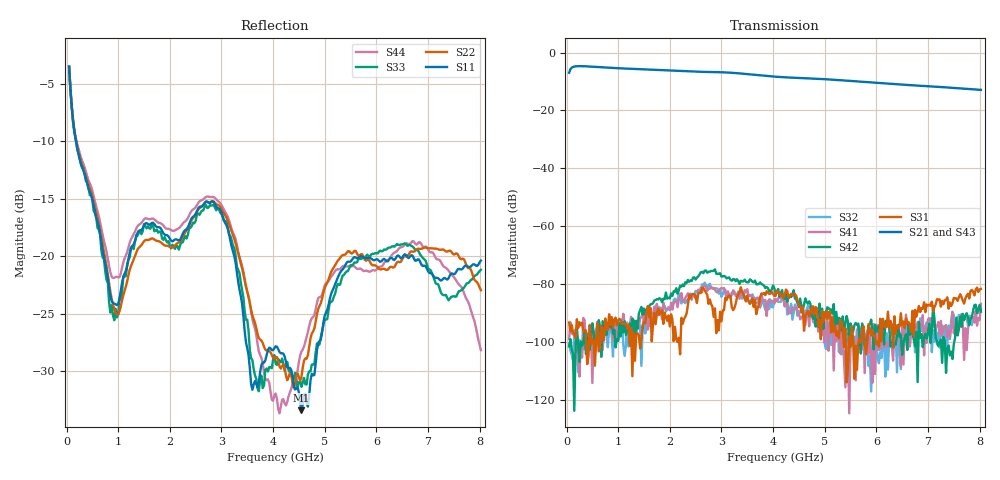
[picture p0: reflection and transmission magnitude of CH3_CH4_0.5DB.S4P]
!Agilent Technologies,E5071C,MY46316741,A.11.02
!Date: Thu May 28 15:04:49 2026
!Data & Calibration Information:
!1:CH3 INPUT 2:CH3 OUTPUT 3:CH4 INPUT 4:CH4 OUTPUT
!Freq	S11:SOLT4(ON)	S12:SOLT4(ON)	S13:SOLT4(ON)	S14:SOLT4(ON)
!	S21:SOLT4(ON)	S22:SOLT4(ON)	S23:SOLT4(ON)	S24:SOLT4(ON)
!	S31:SOLT4(ON)	S32:SOLT4(ON)	S33:SOLT4(ON)	S34:SOLT4(ON)
!	S41:SOLT4(ON)	S42:SOLT4(ON)	S43:SOLT4(ON)	S44:SOLT4(ON)
!PortZ  Port1:50+j0  Port2:50+j0  Port3:50+j0  Port4:50+j0
!Above PortZ is port z conversion or system Z0 setting when saving the data.
!When reading, reference impedance value at option line is always used.
# Hz S dB R 50
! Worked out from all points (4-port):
!   320 points, 50 MHz to 8.025 GHz, reference 50 ohm
!   strongest paths, dB at 50 MHz, 2.05 GHz, 4.05 GHz, 6.05 GHz, 8.025 GHz:
!     S21: -7.0, -6.3, -8.3, -10.5, -12.9
!     S43: -6.9, -6.3, -8.4, -10.6, -13.0
!     S31: -93.3, -92.3, -84.0, -101.5, -81.7
!     S42: -101.5, -84.1, -83.3, -94.3, -89.6
!     S41: -99.0, -88.8, -85.1, -102.8, -86.8
!     S32: -100.5, -88.5, -85.2, -107.3, -88.4
!   lowest |S11| = -33.4 dB at 4.55 GHz (marker M1), VSWR 1.04, Z = 49.6 - j2.09 ohm
!   |S11| at or under -10 dB: 181.2 MHz to end of sweep
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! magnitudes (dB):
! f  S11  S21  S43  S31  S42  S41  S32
! 50 MHz  -3.5  -7.0  -6.9  -93.3  -101.5  -99.0  -100.5
! 925 MHz  -24.1  -5.3  -5.4  -92.2  -95.8  -96.0  -93.6
! 2.85 GHz  -15.3  -6.7  -6.8  -91.3  -75.3  -81.4  -81.5
! 4.125 GHz  -28.3  -8.4  -8.5  -83.5  -84.4  -84.2  -86.1
! 4.55 GHz  -33.4  -8.8  -8.9  -89.8  -88.0  -91.4  -89.4
! 5.425 GHz  -20.6  -9.7  -9.8  -114.0  -91.0  -100.6  -96.9
! 8.025 GHz  -20.4  -12.9  -13.0  -81.7  -89.6  -86.8  -88.4
